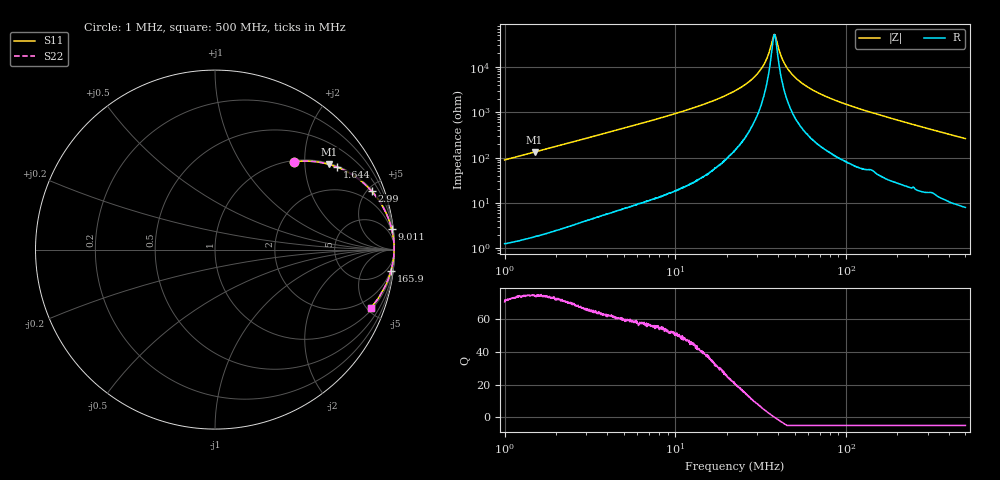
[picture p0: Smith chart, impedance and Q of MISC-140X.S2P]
!s-Parameter Generated by FASTRON Sdn. Bhd.
!FASTRON P/N : MISC-140X
!Keysight Technologies,E4991B,MY54100416,A.01.15
!Date: Mon Mar 16 10:35:19 2026
!Version  : Rev00 Mon Mar 16 10:35:19 2026
!Data & Calibration Information:
!PortZ  Port1:50+j0  Port2:50+j0
!When reading, reference impedance value at option line is always used.
!Remarks : This data is being provided solely for informational purposes.
!Freq	S11	S21	S12	S22
# Hz S dB R 50
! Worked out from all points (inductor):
!   1601 points, 1 MHz to 500 MHz, reference 50 ohm
!   read as one part in series: L = 14.1 uH near 1.032 MHz
!   highest Q = 74.8 at 1.498 MHz (marker M1), where L = 14.1 uH
!   self-resonance near 38.07 MHz
!   S11 on the Smith chart (normalised r, x): 1 MHz: 1.03, +1.78; 1.644 MHz: 1.04, +2.92; 2.99 MHz: 1.08, +5.31; 9.011 MHz: 1, +17; 165.9 MHz: 2, -17; 500 MHz: 1.16, -5.27
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1000000  -3.61 47.9  -2.59 -41.3  -2.59 -41.3  -3.61 47.9
1497728  -2.00 36.6  -4.48 -52.6  -4.48 -52.6  -2.00 36.6
1644060  -1.72 34.2  -5.01 -55.1  -5.01 -55.1  -1.72 34.2
2820919  -0.69 21.6  -8.67 -67.5  -8.67 -67.5  -0.69 21.6
2990153  -0.62 20.5  -9.11 -68.6  -9.11 -68.6  -0.62 20.5
7957584  -0.10 7.8  -17.36 -81.2  -17.36 -81.2  -0.10 7.8
9010744  -0.08 6.8  -18.53 -82.1  -18.53 -82.1  -0.08 6.8
2.236068e7  -0.02 1.9  -29.53 -85.3  -29.53 -85.3  -0.02 1.9
2.715362e7  -0.02 1.2  -33.70 -84.1  -33.70 -84.1  -0.02 1.2
3.122875e7  -0.02 0.7  -38.38 -81.2  -38.38 -81.2  -0.02 0.7
3.414698e7  -0.02 0.4  -43.38 -74.0  -43.38 -74.0  -0.02 0.4
3.719317e7  -0.02 0.1  -52.65 -37.3  -52.65 -37.3  -0.02 0.1
3.807013e7  -0.02 0.0  -54.41 -0.4  -54.41 -0.4  -0.02 0.0
3.896776e7  -0.02 -0.1  -52.49 34.9  -52.49 34.9  -0.02 -0.1
4.227946e7  -0.02 -0.4  -43.64 71.7  -43.64 71.7  -0.02 -0.4
4.587261e7  -0.02 -0.6  -38.91 78.9  -38.91 78.9  -0.02 -0.6
5.234877e7  -0.02 -1.1  -34.27 82.3  -34.27 82.3  -0.02 -1.1
6.307767e7  -0.03 -1.8  -30.11 83.7  -30.11 83.7  -0.03 -1.8
9.265618e7  -0.04 -3.4  -24.50 83.4  -24.50 83.4  -0.04 -3.4
1.659216e8  -0.11 -6.8  -18.48 80.6  -18.48 80.6  -0.11 -6.8
1.77937e8  -0.12 -7.4  -17.82 80.2  -17.82 80.2  -0.12 -7.4
5e8  -0.67 -20.5  -9.09 67.7  -9.09 67.7  -0.67 -20.5
